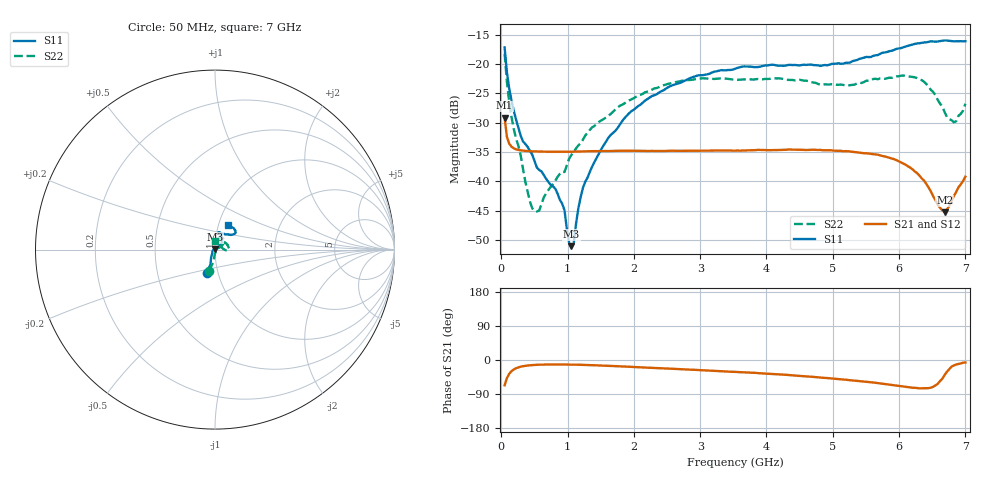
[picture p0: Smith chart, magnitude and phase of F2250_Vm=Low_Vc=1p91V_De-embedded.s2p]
! Integrated Device Technology
! Corporate Headquarters
! 6024 Silver Creek Valley Road
! San Jose, CA 95138  USA
! Phone:  1-408-284-8200
! Toll Free:  1-800-223-1366
! Webpage:  http://www.idt.com/
! Timing and RF Division
! 515 Groton Road, Suite 102
! Westford, MA 01886-6024
! Device:  F2250
! Description: Voltage Variable RF Attenuator
! Frequency:  50.0 -  6000.00 MHz
! Package:  3x3 mm Thin QFN Plastic Package: 16 pin
! Ports:  2 RF, 3 DC
!  Pin  1  = GND
!  Pin  2  = NC
!  Pin  3  = RF1  = Port 1
!  Pin  4  = NC
!  Pin  5  = GND
!  Pin  6  = GND
!  Pin  7  = GND
!  Pin  8  = GND
!  Pin  9  = NC
!  Pin 10  = RF2  = Port 2
!  Pin 11  = NC
!  Pin 12  = GND
!  Pin 13  = GND
!  Pin 14  = VCNTRL
!  Pin 15  = VDD
!  Pin 16  = VMODE
! Vcntrl:  1.910 Volts
! Vmode:  +0.000 Volts
! Vdd:  +3.30  Volts
! Current:  1.183 mA
! Data:  The device was measured on a the F2250 evaluation board which has
!  individual transmission lines to the RF pins.  Data was collected
!  using a calibrated network analyzer.  The evaluation board was
!  de-embedded using a TRL calibration technique.
!  The reference plane is the edge of the package pin.
! Misc:  SN 10
!  Action Tracker AT0258
! Date Measured:  2014-11-26
! Date:  2015-10-15  MJV
! Note:
!  Integrated Device Technology supplies this data as a sample of measured
!  data at the package pin for this product.  Your particular data for this
!  product may vary.
!  Data was taken at 25 degrees C.
!  Integrated Device Technology reserves the right to change this data at anytime.
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# GHz S dB R 50
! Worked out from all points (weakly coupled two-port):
!   201 points, 50 MHz to 7 GHz, reference 50 ohm
!   highest |S21| = -29.13 dB at 50 MHz (marker M1); lowest = -45.2 dB at 6.687 GHz (marker M2)
!   lowest |S11| = -51.0 dB at 1.058 GHz (marker M3), VSWR 1.01, Z = 49.9 + j0.24 ohm
!   |S11| at or under -10 dB: start of sweep to end of sweep
!   |S22| runs from -45.1 to -18.2 dB; largest |S21 - S12| = 6.6e-05
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0.05  -17.18 -108.5  -29.13 -66.8  -29.13 -66.8  -18.24 -105.9
0.08475  -21.44 -107.3  -32.40 -47.7  -32.40 -47.7  -23.03 -97.5
0.189  -28.01 -119.4  -34.36 -24.9  -34.36 -24.9  -31.09 -93.5
0.328  -33.19 -133.4  -34.75 -16.4  -34.76 -16.4  -37.89 -73.9
0.467  -35.45 -146.9  -34.86 -13.4  -34.86 -13.4  -44.56 -36.4
0.57125  -38.04 -160.2  -34.90 -12.4  -34.90 -12.4  -44.96 -9.1
0.91875  -43.78 157.8  -34.94 -11.9  -34.94 -11.9  -38.33 21.5
0.9535  -44.91 170.2  -34.94 -11.9  -34.95 -11.9  -38.39 28.2
1.023  -50.45 143.4  -34.94 -12.0  -34.93 -12.0  -36.13 28.4
1.05775  -51.01 121.3  -34.93 -12.1  -34.93 -12.1  -35.48 29.5
1.0925  -50.52 87.1  -34.92 -12.2  -34.92 -12.2  -34.99 28.1
1.162  -44.57 55.2  -34.91 -12.5  -34.90 -12.5  -33.87 25.1
1.2315  -41.08 43.3  -34.87 -12.8  -34.88 -12.8  -32.89 23.3
1.61375  -32.59 40.6  -34.82 -15.4  -34.81 -15.3  -28.84 30.4
2.37825  -24.87 47.2  -34.79 -21.5  -34.79 -21.6  -23.94 38.1
3.525  -20.81 72.4  -34.75 -31.3  -34.75 -31.4  -22.68 63.9
4.7065  -20.18 72.3  -34.60 -44.6  -34.60 -44.6  -23.15 65.8
5.85325  -17.82 40.4  -35.96 -65.0  -35.96 -65.1  -22.33 12.1
6.33975  -16.41 40.9  -39.44 -74.7  -39.45 -74.8  -22.75 -2.0
6.68725  -15.99 48.8  -45.23 -39.4  -45.20 -39.0  -28.20 18.0
6.82625  -16.14 53.5  -42.48 -14.4  -42.46 -14.3  -29.93 51.8
7  -16.13 63.2  -39.17 -6.6  -39.12 -6.7  -26.75 91.8
